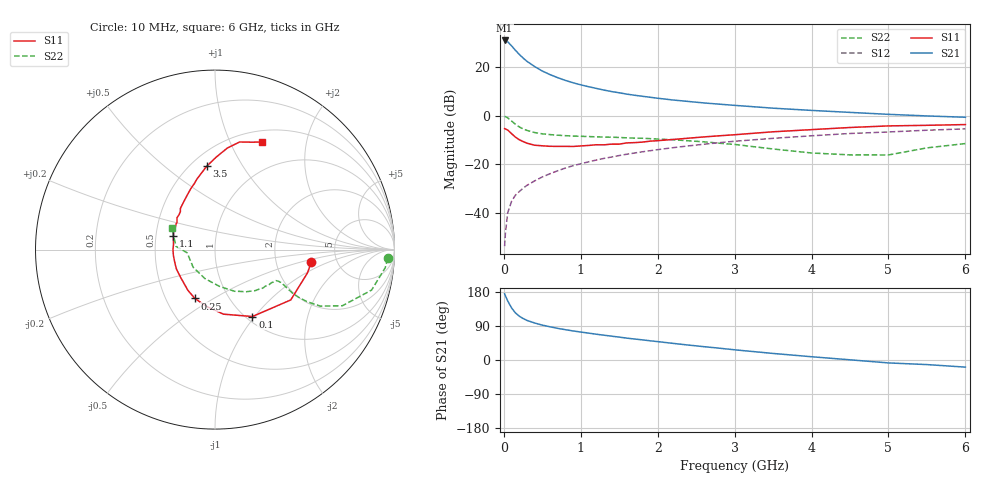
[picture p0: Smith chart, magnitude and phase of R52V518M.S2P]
! SIEMENS Small Signal Semiconductors
! BFR183
! Si NPN RF Bipolar Junction Transistor in SOT23
! VCE = 2.5 V  IC = 18 mA
! Common Emitter S-Parameters:  May  1996
# GHz  S  MA  R  50
!  f  S11  S21  S12  S22
! GHz  MAG  ANG  MAG  ANG  MAG  ANG  MAG  ANG
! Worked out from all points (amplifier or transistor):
!   36 points, 10 MHz to 6 GHz, reference 50 ohm
!   highest |S21| = 30.8 dB at 10 MHz (marker M1)
!   |S21| within 3 dB of that: start of sweep to 122.2 MHz
!   unconditionally stable (mu >= 1): 557.9 MHz to 2.37 GHz
!   at 250 MHz: K = 0.79, MSG = 26.7 dB, |S12| = -29.8 dB
!   at 1.4 GHz: K = 1.05, MAG = 12.1 dB, |S12| = -17.0 dB
!   at 6 GHz: K = 0.90, MSG = 2.4 dB, |S12| = -5.4 dB
!   S11 on the Smith chart (normalised r, x): 10 MHz: 3.22, -0.63; 100 MHz: 1.07, -0.97; 250 MHz: 0.70, -0.42; 1.1 GHz: 0.62, +0.10; 3.5 GHz: 0.60, +0.71; 6 GHz: 0.63, +1.33
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0.01  0.5411 -7.3  34.8 174.8  0.0021 88.2  0.9638 -2.9
0.02  0.5315 -14.1  34.64 169.7  0.0038 87.1  0.9537 -6.1
0.05  0.5067 -33.6  32.65 155.9  0.0101 78.3  0.9011 -14.5
0.1  0.4272 -60.8  27.04 137.7  0.0174 72.6  0.7755 -23.8
0.15  0.3627 -82.6  21.92 124.4  0.0233 66.9  0.6667 -28.2
0.2  0.3204 -98.2  18.1 115.8  0.0276 67.5  0.5881 -29.5
0.25  0.2944 -112.4  15.18 109.5  0.0324 66.8  0.5342 -29.7
0.3  0.2722 -123.8  13.02 104.5  0.0371 67.8  0.4979 -29.4
0.4  0.2466 -140.7  10.14 97.7  0.0458 69.6  0.4501 -27.9
0.5  0.2404 -153.7  8.207 92.0  0.0552 70.3  0.4227 -26.9
0.6  0.2346 -164.2  6.938 87.6  0.0643 70.6  0.4081 -26.5
0.7  0.234 -172.3  6.004 83.5  0.0739 70.8  0.3968 -26.5
0.8  0.2341 179.7  5.277 80.0  0.0841 70.0  0.3879 -26.7
0.9  0.2329 172.8  4.719 76.7  0.0938 70.0  0.3807 -27.0
1.1  0.2444 161.8  3.922 71.0  0.1126 68.8  0.3721 -29.0
1.3  0.2516 152.1  3.342 65.5  0.1325 67.3  0.3635 -31.0
1.6  0.2759 140.1  2.758 57.7  0.1616 64.7  0.3499 -35.2
2.2  0.3242 121.4  2.089 43.9  0.22 58.4  0.3201 -45.6
3.5  0.466 95.8  1.421 17.3  0.3419 42.1  0.2068 -82.8
4.5  0.5706 83.0  1.164 0.5  0.4299 29.4  0.1566 -141.0
5.5  0.6325 71.1  0.985 -12.1  0.5017 17.5  0.2178 175.3
6  0.655 66.2  0.925 -18.8  0.5352 9.8  0.2672 153.8
